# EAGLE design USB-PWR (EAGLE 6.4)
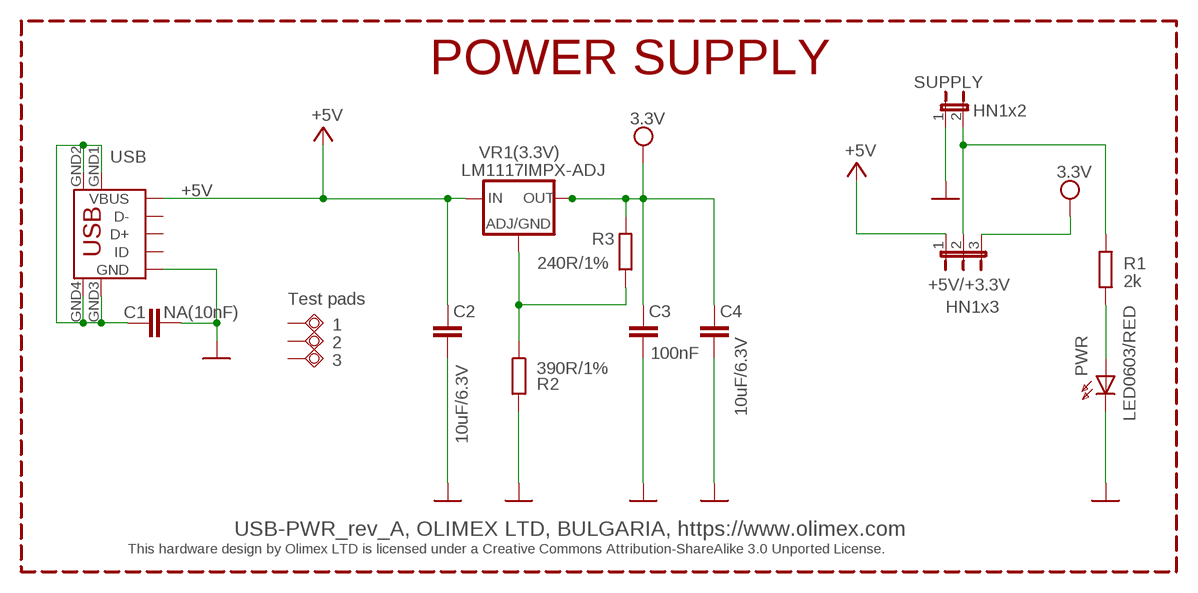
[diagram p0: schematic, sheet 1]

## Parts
1  TESTPAD40/70  [TESTPAD]
2  TESTPAD40/70  [TESTPAD]
3  TESTPAD40/70  [TESTPAD]
+5V/+3.3V  HN1x3  JP2E  [JP2]
C1  NA(10nF)  C-EUC0603_5MIL  [C0603_5MIL]
C2  10uF/6.3V  C-EUC0603_5MIL  [C0603_5MIL]
C3  100nF  C-EUC0603_5MIL  [C0603_5MIL]
C4  10uF/6.3V  C-EUC0603_5MIL  [C0603_5MIL]
PWR  LED0603/RED  LED0603DWS  [LED-0603]
R1  2k  R-EU_R0603_5MIL  [R0603_5MIL]
R2  390R/1%  R-EU_R0603_5MIL  [R0603_5MIL]
R3  240R/1%  R-EU_R0603_5MIL  [R0603_5MIL]
SUPPLY  HN1x2  JP1E  [JP1]
USB  USB-OTG  MINI_USB9  [USB_MINI_9PIN]
VR1(3.3V)  LM1117IMPX-ADJ  LM1117  [SOT223]

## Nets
+5V: +5V/+3.3V.1 C2.1 USB.VBUS VR1(3.3V).3(IN)
GND [pwr]: C1.1 C2.2 C3.2 C4.2 PWR.C R2.2 SUPPLY.1 USB.GND
N$2: +5V/+3.3V.2 R1.2 SUPPLY.2
N$16: PWR.A R1.1
N$100: R2.1 R3.1 VR1(3.3V).1(ADJ/GND)
USB_SHIELD1: C1.2 USB.GND1 USB.GND2 USB.GND3 USB.GND4
VCC: +5V/+3.3V.3 C3.1 C4.1 R3.2 VR1(3.3V).2(OUT) VR1(3.3V).4(RAD) ; supply symbol labelled 3.3V
Unconnected: 1.P$1(PP) 2.P$1(PP) 3.P$1(PP) USB.D+ USB.D- USB.ID

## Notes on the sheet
- POWER SUPPLY
- Test pads
- USB-PWR_rev_A, OLIMEX LTD, BULGARIA, https://www.olimex.com
- This hardware design by Olimex LTD is licensed under a Creative Commons Attribution-ShareAlike 3.0 Unported License.

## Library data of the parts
1-3 = gogo:TESTPAD: drill 40mils, diameter 70mils
+5V/+3.3V = jumper:JP2E: JUMPER
C1-C4 = rcl:C-EU: CAPACITOR, European symbol
PWR = DOUBLE-SIDE:LED
R1-R3 = rcl:R-EU_: RESISTOR, European symbol
SUPPLY = jumper:JP1E: JUMPER
USB = OLIMEX_CONNECTORS:MINI_USB9
VR1(3.3V) = arm:LM1117

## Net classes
1 pwr: width 0.201 mm, clearance 0.201 mm

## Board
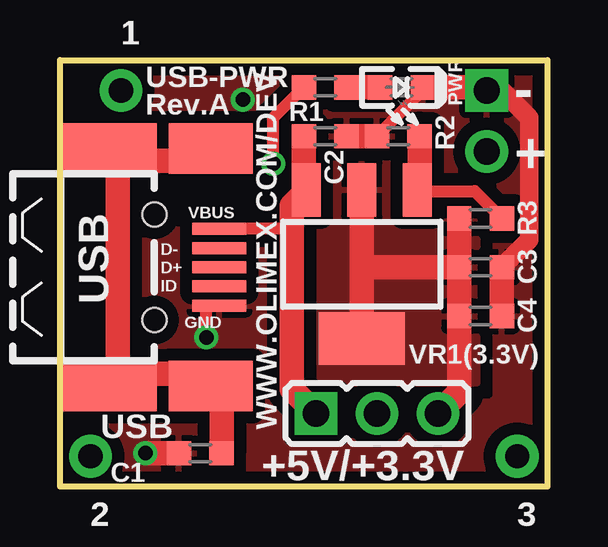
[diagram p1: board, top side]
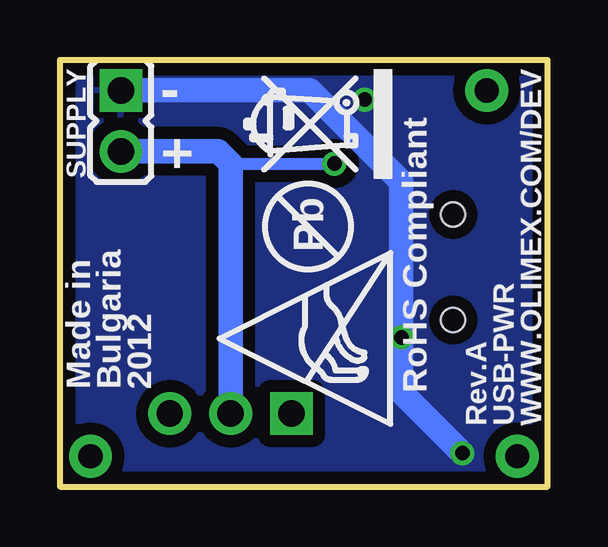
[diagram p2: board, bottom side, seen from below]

Size 20.32 x 17.78 mm. Coordinates in mm from the lower left corner, seen from the top.
Outline: 20.32,0 0,0 0,17.78 20.32,17.78 20.32,0
Copper layers (1+16): Top 0.035mm / dielectric 1.5mm / Bottom 0.035mm
Design rules "default": minimum track width 8mil, minimum drill 15mil, track to track 8mil, track to pad 8mil, pad to pad 8mil, via to via 8mil, smd to smd 8mil, copper to edge 10mil, drill to drill 8mil, minimum pad ring 10mil, minimum via ring 8mil, stop-mask expansion 4mil, vias tented up to drill 25mil, thermal gap 10mil

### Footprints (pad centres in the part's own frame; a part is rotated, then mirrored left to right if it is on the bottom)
TESTPAD = drill 1.016 pad 1.778: P$1 0,0
JP2 = drill 1.1 pad 1.778 square: 1 -2.54,0 | drill 1.1 pad 1.778: 2 0,0; 3 2.54,0
C0603_5MIL = smd 1.016 x 1.016: 1 -0.889,0; 2 0.889,0
LED-0603 = smd 1.016 x 1.016: A 0.889,0; C -0.889,0
R0603_5MIL = smd 1.016 x 1.016: 1 -0.889,0; 2 0.889,0
JP1 = drill 1.1 pad 1.778 square: 1 0,-1.27 | drill 1.1 pad 1.778: 2 0,1.27
USB_MINI_9PIN = smd 2.25 x 0.5: D+ 2.706,0; D- 2.706,0.8; GND 2.706,-1.6; ID 2.706,-0.8; VBUS 2.706,1.6 | smd 4 x 2.1: GND1 -1.9,4.95; GND3 -1.9,-4.95 | smd 3.5 x 2.1: GND2 2.35,4.95; GND4 2.35,-4.95 | hole 1: 0,2.2; 0,-2.2
SOT223 = smd 1.219 x 2.235: 1 -2.311,-3.099; 2 0,-3.099; 3 2.311,-3.099 | smd 3.6 x 2.2: 4 0,3.099

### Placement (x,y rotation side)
1  2.54,16.51 0 top
2  1.27,1.27 0 top
3  19.05,1.27 0 top
+5V/+3.3V  13.21,3.05 0 top
C1  5.84,1.4 0 top
C2  11.05,14.61 0 top
C3  17.53,9.14 0 top
C4  17.53,7.11 0 top
PWR  14.22,16.64 180 top
R1  11.05,16.64 180 top
R2  14.1,14.61 180 top
R3  17.53,11.18 180 top
SUPPLY  17.78,15.24 180 bottom
U$1  [ESD_SYMBOL]  6.55,2.62 90 bottom
U$2  [RECYCLE_BIN1/8]  6.48,12.83 90 bottom
U$7  [PB_SMALL]  9.98,10.85 90 bottom
USB  3.94,9.14 0 top
VR1(3.3V)  12.57,9.27 180 top

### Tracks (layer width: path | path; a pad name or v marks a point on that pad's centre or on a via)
+5V
  Top 0.508: USB.VBUS 9.35,10.74 10.13,11.53 10.13,12.19 10.13,12.37 VR1(3.3V).3
  Top 1.016: VR1(3.3V).3 10.16,12.47 C2.1 | +5V/+3.3V.1 9.65,4.06 9.65,11.71 10.13,12.19 10.16,12.19
GND  (via drill 0.6)
  Top 0.508: R2.2 15.11,16.51 PWR.C | USB.GND 6.1,7.54 v6.1,6.22
  Top 0.762: C3.2 19.56,10.29 19.56,15.37 18.41,16.51 SUPPLY.1
  Top 1.016: R2.2 C2.2 | C3.2 C4.2 | C1.1 v3.56,1.4 | SUPPLY.1 17.65,16.64 PWR.C
  Bottom 1.016: v3.56,1.4 6.1,3.94 v6.1,6.22 6.1,12.7 9.91,16.51 SUPPLY.1
  other vias: 7.62,16.13
  pour Bottom (isolate 0.508, rank 2): -2.54,-2.54 22.86,-2.54 22.86,20.32 -2.54,20.32
  pour Top (isolate 0.508, rank 2): -5.08,-5.08 25.4,-5.08 25.4,22.86 -5.08,22.86
N$2  (via drill 0.6)
  Top 0.508: R1.2 8.89,15.37 v8.89,13.46
  Bottom 0.508: 13.21,13.46 v8.89,13.46
  Bottom 1.016: +5V/+3.3V.2 13.21,13.46 13.72,13.97 SUPPLY.2
N$16
  Top 1.016: R1.1 PWR.A
N$100
  Top 0.508: R3.1 17.27,12.32 15.14,12.32 14.99,12.47
  Top 1.016: VR1(3.3V).1 14.99,12.47 R2.1
USB_SHIELD1
  Top 1.016: USB.GND2 6.29,13.59 2.41,13.59 | USB.GND1 2.04,13.59 2.41,13.59 | USB.GND3 2.04,4.7 2.41,4.7 | 2.41,4.7 2.41,13.59 | 2.41,4.7 6.29,4.7 USB.GND4 6.73,4.19 C1.2
VCC
  Top 1.016: C3.1 C4.1 16.64,3.94 +5V/+3.3V.3 | VR1(3.3V).4 12.57,9.14 | 12.57,9.14 VR1(3.3V).2 | 12.57,9.14 C3.1 | C3.1 R3.2
  pour Top (isolate 0.508): 11.05,13.84 11.05,12.32 11.05,10.92 10.41,10.92 10.41,4.32 15.88,4.32 17.4,4.32 17.4,11.05 14.1,11.05 14.1,13.84 11.3,13.84

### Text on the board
tNames: USB-PWR | - | Rev.A | + | WWW.OLIMEX.COM/DEV
bNames: - | RoHS Compliant | + | 2012 | Bulgaria | Made in | WWW.OLIMEX.COM/DEV | USB-PWR | Rev.A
